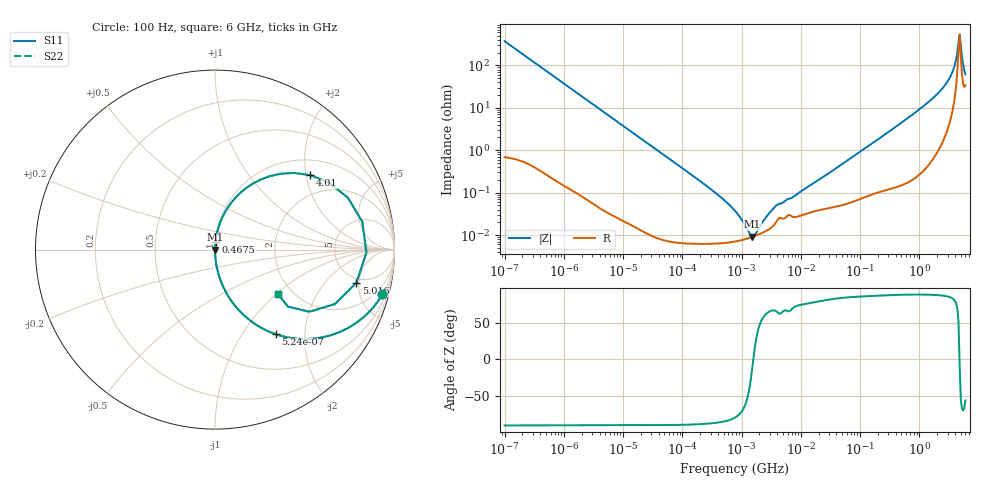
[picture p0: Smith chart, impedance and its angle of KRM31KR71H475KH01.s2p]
!Murata Part Number: KRM31KR71H475KH01
!These Parameters are Measured in Series Mode Connection
!Data Generated on Jan 08, 2026
!  o--ll--o
!Port1  Port2
!  o------o
!Operation Temp=25[degC], DC Bias Voltage=0[V]
!Freq. Start=100[Hz] Stop=6[GHz] 401[Steps]
# Hz S RI R 50
!Freq.(Hz) S11(Real) S11(Imag) S21(Real) S21(Imag) S12(Real) S12(Imag) S22(Real) S22(Imag)
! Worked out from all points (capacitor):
!   401 points, 100 Hz to 6 GHz, reference 50 ohm
!   read as one part in series: C = 4.25 uF near 109 Hz
!   lowest |Z| = 9.23 mohm at 1.516 MHz (marker M1)
!   series resonance near 1.577 MHz, so ESL is about 2.4 nH
!   S11 on the Smith chart (normalised r, x): 100 Hz: 1.01, -7.48; 524 Hz: 1.01, -1.43; 467.5 MHz: 1.00, +0.08; 4.01 GHz: 1.39, +2.12; 5.016 GHz: 4.37, -4.68; 6 GHz: 1.69, -1.02
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100  0.9329 -0.2493  0.0671 0.2493  0.0671 0.2493  0.9329 -0.2493
205  0.7693 -0.4198  0.2307 0.4198  0.2307 0.4198  0.7693 -0.4198
524  0.3395 -0.4718  0.6605 0.4718  0.6605 0.4718  0.3395 -0.4718
981  0.129 -0.3332  0.871 0.3332  0.871 0.3332  0.129 -0.3332
2008  0.0347 -0.1809  0.9653 0.1809  0.9653 0.1809  0.0347 -0.1809
6433  0.00373 -0.0585  0.9963 0.0585  0.9963 0.0585  0.00373 -0.0585
40335  0.00017 -0.0094  0.9998 0.0094  0.9998 0.0094  0.00017 -0.0094
330837  6.38e-05 -0.00109  0.9999 0.00109  0.9999 0.00109  6.38e-05 -0.00109
774597  7.04e-05 -0.000367  0.9999 0.000367  0.9999 0.000367  7.04e-05 -0.000367
1516199  9.05e-05 -1.81e-05  0.9999 1.81e-05  0.9999 1.81e-05  9.05e-05 -1.81e-05
1734173  9.71e-05 4.38e-05  0.9999 -4.38e-05  0.9999 -4.38e-05  9.71e-05 4.38e-05
3882480  0.000208 0.000456  0.9998 -0.000456  0.9998 -0.000456  0.000208 0.000456
1.555665e7  0.000353 0.00156  0.9996 -0.00156  0.9996 -0.00156  0.000353 0.00156
3.124326e8  0.00198 0.0278  0.998 -0.0278  0.998 -0.0278  0.00198 0.0278
4.674818e8  0.00317 0.0415  0.9968 -0.0415  0.9968 -0.0415  0.00317 0.0415
2.450438e9  0.0869 0.2564  0.9131 -0.2564  0.9131 -0.2564  0.0869 0.2564
3.205649e9  0.2118 0.3681  0.7882 -0.3681  0.7882 -0.3681  0.2118 0.3681
4.009986e9  0.5311 0.4148  0.4689 -0.4148  0.4689 -0.4148  0.5311 0.4148
4.586474e9  0.8208 0.1553  0.1792 -0.1553  0.1792 -0.1553  0.8208 0.1553
5.016141e9  0.7881 -0.1845  0.2119 0.1845  0.2119 0.1845  0.7881 -0.1845
5.486059e9  0.526 -0.3464  0.474 0.3464  0.474 0.3464  0.526 -0.3464
6e9  0.3493 -0.2459  0.6507 0.2459  0.6507 0.2459  0.3493 -0.2459
